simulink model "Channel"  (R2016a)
settings: Solver=ode3  StartTime=0.0  StopTime=6  FixedStep=1/5000000  RelTol=1e-3
libraries: commchan3 x2

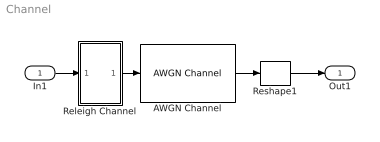
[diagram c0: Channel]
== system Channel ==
  In1 : Inport
  AWGN Channel : commchan3/AWGN Channel  InputProcessing=Columns as channels (frame based)  seed=67  noiseMode="Signal to noise ratio  (Eb/No)"  EbNodB=10  EsNodB=10  SNRdB=10  bitsPerSym=2  Ps=1  Tsym=1/5000000  variance=1
  Releigh Channel : Subsystem
  Reshape1 : Reshape
  Out1 : Outport
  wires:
  Releigh Channel/1(Out1) -> AWGN Channel/1
  In1/1 -> Releigh Channel/1(In1)
  AWGN Channel/1 -> Reshape1/1
  Reshape1/1 -> Out1/1

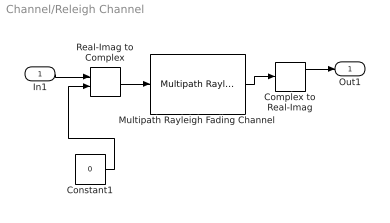
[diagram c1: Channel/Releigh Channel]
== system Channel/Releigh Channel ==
  In1 : Inport
  Complex to Real-Imag : ComplexToRealImag
  Constant1 : Constant  Value=0  SampleTime=1/5000000
  Multipath Rayleigh Fading Channel : commchan3/Multipath Rayleigh Fading Channel  maxDopplerShift=1  spectrumType=Jakes  sigmaGaussian=1/sqrt(2)  coeffRounded=[1 -1.72 0.785]  freqMinMaxRJakes=[0 1]  freqMinMaxAJakes=[0 1]  sigmaGaussian1=1/sqrt(2)  sigmaGaussian2=1/sqrt(2)  centerFreqGaussian1=0.0  centerFreqGaussian2=0.0  gainGaussian1=0.5  gainGaussian2=0.5  coeffBell=9  dopplerSpectrum=doppler.jakes  pathDelays=0  avgPathGaindB=-3  normalizePathGains=on  seed=73  enableProbe=0  openVisAtStart=off  outPathGains=off  outDelay=off
  Real-Imag to Complex : RealImagToComplex
  Out1 : Outport
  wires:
  Real-Imag to Complex/1 -> Multipath Rayleigh Fading Channel/1
  Multipath Rayleigh Fading Channel/1 -> Complex to Real-Imag/1
  Constant1/1 -> Real-Imag to Complex/2
  Complex to Real-Imag/1 -> Out1/1
  Complex to Real-Imag/2 -> ?
  In1/1 -> Real-Imag to Complex/1
